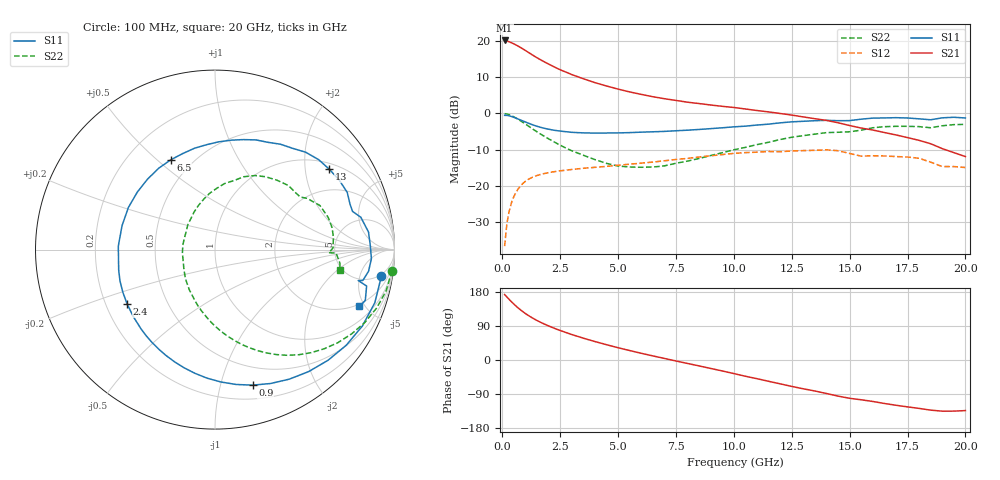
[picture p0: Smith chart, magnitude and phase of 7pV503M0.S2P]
! Infineon Technologies  Discrete & RF Semiconductors
! bfp620
! VCE = 0.50 V,  IC =  3.0 mA
! Common Emitter S-Parameters:  Sep 2002
# GHz  S  MA  R  50
!  f  S11  S21  S12  S22
! GHz  MAG  ANG  MAG  ANG  MAG  ANG  MAG  ANG
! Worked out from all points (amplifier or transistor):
!   59 points, 100 MHz to 20 GHz, reference 50 ohm
!   highest |S21| = 20.1 dB at 100 MHz (marker M1)
!   |S21| within 3 dB of that: start of sweep to 1.056 GHz
!   unconditionally stable (mu >= 1): 5.341 GHz to 11.46 GHz; 14.92 GHz to 15.23 GHz; 17.03 GHz to end of sweep
!   at 1 GHz: K = 0.24, MSG = 18.0 dB, |S12| = -18.7 dB
!   at 5.5 GHz: K = 1.02, MAG = 9.2 dB, |S12| = -14.0 dB
!   at 20 GHz: K = 1.90, MAG = -3.9 dB, |S12| = -14.9 dB
!   S11 on the Smith chart (normalised r, x): 100 MHz: 4, -11; 900 MHz: 0.32, -1.26; 2.4 GHz: 0.29, -0.26; 6.5 GHz: 0.38, +0.55; 13 GHz: 1.19, +2.69; 20 GHz: 1.84, -4.59
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0.1  0.9391 -9.0  10.12 172.7  0.0148 83.2  0.9926 -6.8
0.2  0.9384 -18.4  9.941 166.2  0.0307 79.6  0.9809 -13.5
0.3  0.925 -27.4  9.69 159.7  0.0454 74.3  0.9581 -19.8
0.5  0.8814 -44.4  9.077 147.6  0.0714 64.5  0.8948 -31.6
0.7  0.832 -60.2  8.397 136.6  0.0925 55.9  0.8223 -42.2
0.9  0.7837 -74.5  7.697 127.0  0.1091 48.7  0.7487 -51.5
1.2  0.7177 -93.5  6.693 114.7  0.1271 39.9  0.645 -63.3
1.5  0.6644 -109.9  5.843 104.2  0.1393 33.1  0.5569 -73.3
1.9  0.6145 -128.5  4.97 92.6  0.1504 26.4  0.4656 -84.5
2.4  0.5757 -148.2  4.132 80.1  0.1601 20.0  0.3792 -97.1
3  0.5483 -168.2  3.426 67.2  0.1687 14.0  0.3055 -111.5
3.5  0.539 177.9  3.003 57.6  0.1752 10.1  0.265 -122.8
5  0.5385 143.4  2.162 32.4  0.1929 0.9  0.1883 -160.3
6.5  0.5577 116.3  1.698 10.8  0.2134 -7.5  0.1822 159.4
7  0.5647 108.4  1.594 4.2  0.2223 -10.3  0.1891 148.1
8.5  0.6006 88.1  1.366 -15.6  0.2505 -20.3  0.2393 119.2
10.5  0.667 63.6  1.15 -42.9  0.2882 -38.2  0.3402 88.7
13  0.7785 35.1  0.894 -76.0  0.3072 -61.7  0.4939 55.3
13.5  0.7929 29.4  0.845 -81.8  0.3099 -66.8  0.5179 48.4
15  0.7955 15.5  0.68 -101.0  0.2803 -87.3  0.5578 31.7
17  0.8729 -3.3  0.505 -119.4  0.2542 -97.9  0.6637 10.6
20  0.8645 -21.4  0.254 -133.5  0.1794 -114.9  0.7054 -9.5
